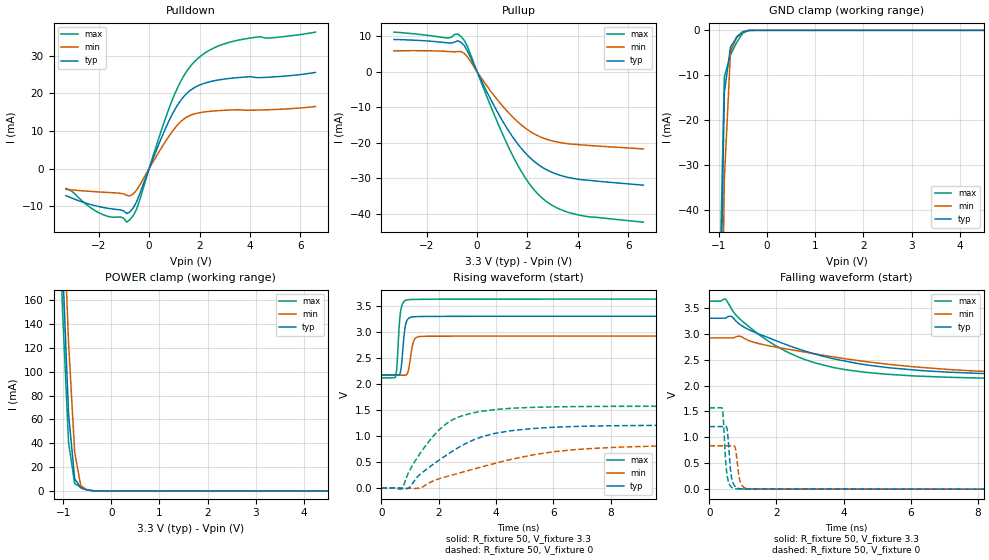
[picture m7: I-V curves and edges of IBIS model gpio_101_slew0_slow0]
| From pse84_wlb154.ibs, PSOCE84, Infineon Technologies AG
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[Model] gpio_101_slew0_slow0
Model_type I/O
Enable   Active-High
Vinl  =  0.99
Vinh  =  2.31
Vmeas =  1.65
Cref  =  15e-12
| Capacitance   typ   min   max
C_comp   1.09946e-12   1.086232e-12   1.114407e-12
| Variables   typ   min   max
[GND Clamp Reference]   0   0   0
[POWER Clamp Reference]   3.3   2.92   3.63
[Pulldown Reference]   0   0   0
[Pullup Reference]   3.3   2.92   3.63
[Temperature Range]   25   125   -40
[Voltage Range]   3.3   2.92   3.63
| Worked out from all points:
|   slope of the pulldown table from 0 to 0.495 V, typ, clamps not added: 59.8 ohm
|   slope of the pullup table from 0 to 0.495 V, typ, clamps not added: 69.5 ohm
|   GND clamp passes 1 mA (typ) near -0.57 V on its own axis
|   POWER clamp passes 1 mA (typ) near -0.52 V on its own axis
|   falling waveform, R_fixture 50, V_fixture 3.3: 20-80 % time 3.54ns typ, 5.22ns min, 2.42ns max; typ from 3.3 V to 2.17 V
|   falling waveform, R_fixture 50, V_fixture 0: 20-80 % time 97ps typ, 105ps min, 92.4ps max; typ from 1.21 V to 0 V
|   rising waveform, R_fixture 50, V_fixture 3.3: 20-80 % time 114ps typ, 135ps min, 103ps max; typ from 2.17 V to 3.3 V
|   rising waveform, R_fixture 50, V_fixture 0: 20-80 % time 2.12ns typ, 3.71ns min, 1.36ns max; typ from 0 V to 1.21 V
[GND Clamp]
| Voltage   I(typ)   I(min)   I(max)
-1.65V    -892.5mA   -911.9mA   -883.9mA
-1.015V   -92.32mA   -129.7mA   -71.28mA
-888.3mV  -13.83mA   -33.21mA   -10.31mA
-761.4mV  -3.792mA   -4.944mA   -5.509mA
-634.5mV  -1.622mA   -1.436mA   -2.707mA
-507.6mV  -326.2uA   -352.3uA   -651.6uA
-380.7mV  -13.48uA   -32.14uA   -19.55uA
-253.8mV  -189.4nA   -1.276uA   -466.7nA
6.6V      0A         0A         0A
[POWER Clamp]
| Voltage   I(typ)   I(min)   I(max)
-1.523V   838.1mA    872.9mA    823.9mA
-1.142V   346.5mA    405.1mA    310.5mA
-1.015V   193mA      257.4mA    153.9mA
-888.3mV  64.97mA    124.9mA    40.96mA
-761.4mV  10.28mA    32.7mA     6.184mA
-634.5mV  2.553mA    4.346mA    3.067mA
-507.6mV  805.9uA    960.7uA    1.159mA
-253.8mV  1.454uA    10.02uA    1.678uA
6.6V      0A         0A         0A
[Pulldown]
| Voltage   I(typ)   I(min)   I(max)
-3.3V     -7.203mA   -5.558mA   -5.309mA
-2.03V    -10.05mA   -6.209mA   -11.63mA
-1.142V   -11mA      -6.584mA   -12.87mA
-888.3mV  -11.97mA   -7.139mA   -14.27mA
-507.6mV  -8.987mA   -5.838mA   -10.98mA
341.4mV   5.791mA    3.893mA    7.243mA
910.3mV   14.34mA    9.777mA    18.1mA
1.366V    19.09mA    13.11mA    24.54mA
1.821V    21.6mA     14.58mA    28.57mA
2.503V    23.23mA    15.27mA    31.85mA
3.3V      24.03mA    15.58mA    33.77mA
6.6V      25.56mA    16.5mA     36.29mA
[Pullup]
| Voltage   I(typ)   I(min)   I(max)
-3.3V     9.072mA    5.875mA    11.15mA
-1.142V   8.101mA    5.689mA    9.493mA
-761.4mV  8.711mA    5.685mA    10.6mA
-634.5mV  8.24mA     5.672mA    9.896mA
-380.7mV  5.841mA    4.169mA    7.086mA
682.8mV   -9.682mA   -6.781mA   -12.13mA
1.479V    -19.03mA   -13.2mA    -24.52mA
2.048V    -23.85mA   -16.55mA   -31.28mA
2.731V    -27.5mA    -18.94mA   -36.43mA
3.3V      -29.17mA   -19.95mA   -38.76mA
4.051V    -30.32mA   -20.54mA   -40.36mA
6.6V      -31.95mA   -21.74mA   -42.36mA
[Ramp]
dV/dt_r   0.724504/2.11629n  0.501635/3.70646n  0.941981/1.35847n
dV/dt_f   0.678582/3.53628n  0.451032/5.2157n  0.908165/2.41982n
R_load = 50
[Falling Waveform]
R_fixture = 50
V_fixture = 3.3
V_fixture_min = 2.92
V_fixture_max = 3.63
| Time   V(typ)   V(min)   V(max)
0s        3.3V       2.92V      3.63V
477.6ps   3.301V     2.92V      3.667V
646.1ps   3.339V     2.92V      3.493V
832.9ps   3.222V     2.951V     3.333V
1.82ns    2.908V     2.762V     2.832V
2.673ns   2.703V     2.666V     2.547V
3.663ns   2.524V     2.557V     2.354V
6.349ns   2.288V     2.35V      2.18V
12.27ns   2.185V     2.203V     2.119V
800ns     2.169V     2.168V     2.116V
[Falling Waveform]
R_fixture = 50
V_fixture = 0
V_fixture_min = 0
V_fixture_max = 0
| Time   V(typ)   V(min)   V(max)
0s        1.208V     836.1mV    1.57V
384.4ps   1.208V     835.9mV    1.551V
525.2ps   1.172V     836.1mV    283.5mV
600.9ps   582.3mV    836.1mV    85.57mV
651.1ps   265.7mV    836.1mV    40.91mV
721ps     95.7mV     839.1mV    16.99mV
784.6ps   40.24mV    760.3mV    8.097mV
911.6ps   9.059mV    163.8mV    3.285mV
1.067ns   3.049mV    20.83mV    2.694mV
800ns     15.83nV    505.1nV    9.038nV
[Rising Waveform]
R_fixture = 50
V_fixture = 3.3
V_fixture_min = 2.92
V_fixture_max = 3.63
| Time   V(typ)   V(min)   V(max)
0s        2.169V     2.168V     2.116V
496ps     2.169V     2.168V     2.151V
544.2ps   2.169V     2.168V     2.371V
648.4ps   2.197V     2.168V     3.306V
699.3ps   2.357V     2.168V     3.479V
762.3ps   2.777V     2.168V     3.566V
881.4ps   3.209V     2.179V     3.612V
1.169ns   3.292V     2.868V     3.624V
1.83ns    3.297V     2.916V     3.628V
800ns     3.3V       2.92V      3.63V
[Rising Waveform]
R_fixture = 50
V_fixture = 0
V_fixture_min = 0
V_fixture_max = 0
| Time   V(typ)   V(min)   V(max)
0s        16.07nV    504.8nV    9.389nV
709.8ps   -8.838mV   39.34uV    -12.39mV
1.063ns   69.83mV    -10.78mV   417.5mV
1.761ns   437.4mV    126.2mV    966.9mV
2.137ns   583.8mV    198.5mV    1.183V
2.75ns    797.7mV    293.2mV    1.376V
4.389ns   1.092V     532.1mV    1.527V
7.929ns   1.196V     775.1mV    1.569V
18.07ns   1.208V     837.2mV    1.57V
800ns     1.208V     836.1mV    1.57V
